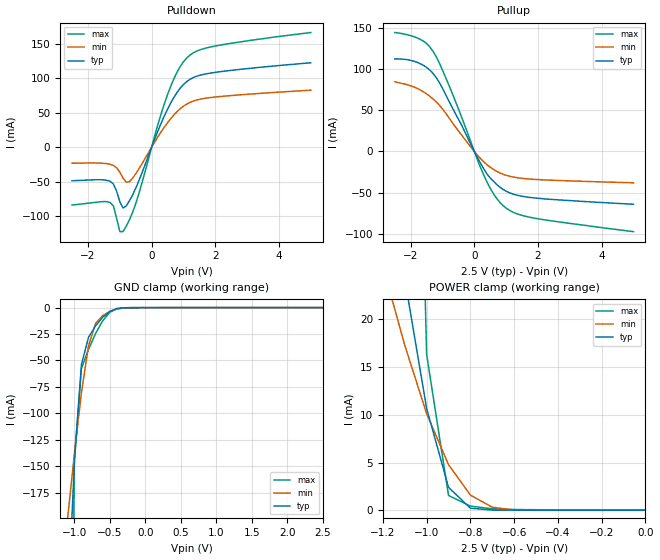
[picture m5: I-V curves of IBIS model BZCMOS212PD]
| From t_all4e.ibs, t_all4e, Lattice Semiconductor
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|   BZCMOS212PD
[Model]   BZCMOS212PD
Model_type   I/O
Polarity   Non-Inverting
Enable   Active-Low
C_comp   2pF   2pF   2pF
Vinl = 0.5
Vinh = 2.64
[Temperature Range]   25.0000   125.0000   -40.0000
[Voltage Range]   2.5000V   2.3000V   2.7000V
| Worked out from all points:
|   slope of the pulldown table from 0 to 0.375 V, typ, clamps not added: 8.75 ohm
|   slope of the pullup table from 0 to 0.375 V, typ, clamps not added: 14.4 ohm
|   GND clamp passes 1 mA (typ) near -0.40 V on its own axis
|   POWER clamp passes 1 mA (typ) near -0.83 V on its own axis
[Pulldown]
|voltage   I(typ)   I(min)   I(max)
-2.5V     -48.8mA    -23.34mA   -84mA
-1.3V     -49.7mA    -24.91mA   -80.43mA
-1.2V     -53.63mA   -26.59mA   -85.64mA
-1V       -79.19mA   -36.36mA   -122.6mA
-900mV    -88.4mA    -44.81mA   -122.7mA
-800mV    -85.34mA   -50.83mA   -115mA
-600mV    -69.53mA   -45.12mA   -94.93mA
500mV     55.24mA    35.55mA    76.37mA
900mV     85.88mA    55.98mA    117.3mA
1.2V      98.44mA    64.96mA    133.6mA
2.1V      109.3mA    73.31mA    147.8mA
5V        122.5mA    82.76mA    166.5mA
[Pullup]
|voltage   I(typ)   I(min)   I(max)
-2.5V     112.7mA    84.9mA     144.8mA
-1.7V     106.9mA    74.88mA    136.5mA
-1.5V     102.3mA    70.1mA     131.4mA
-1.3V     95.06mA    64.02mA    122mA
-1.1V     83.89mA    56.39mA    107.7mA
-700mV    53.9mA     35.54mA    71.28mA
300mV     -21.45mA   -12.87mA   -29.21mA
600mV     -36.24mA   -21.85mA   -51.49mA
900mV     -46.14mA   -27.68mA   -65.82mA
1.3V      -52.82mA   -31.67mA   -75.32mA
1.8V      -56.21mA   -33.75mA   -80.53mA
5V        -64.25mA   -38.14mA   -97.6mA
[GND_clamp]
|voltage   I(typ)   I(min)   I(max)
-2.5V     -2.88A     -1.21A     -25.75A
-1.1V     -296.4mA   -202.8mA   -979.3mA
-1V       -147.6mA   -138.6mA   -143.7mA
-900mV    -53.79mA   -80.42mA   -57.6mA
-800mV    -28.05mA   -35.98mA   -39.41mA
-700mV    -17.1mA    -14.8mA    -24.32mA
-600mV    -8.999mA   -7.523mA   -12.36mA
-500mV    -3.595mA   -3.617mA   -4.359mA
-400mV    -879.6uA   -1.324mA   -818.4uA
-300mV    -134.3uA   -303.2uA   -112.8uA
2.5V      32.9uA     13.5uA     72.78uA
[POWER_clamp]
|voltage   I(typ)   I(min)   I(max)
-2.5V     395.1mA    211mA      2.446A
-1.2V     41.69mA    25.58mA    245.1mA
-1.1V     24.27mA    17.3mA     108.6mA
-1V       10.69mA    10.14mA    16.34mA
-900mV    2.423mA    4.798mA    1.578mA
-800mV    241uA      1.613mA    455.8uA
-700mV    43.59uA    342.3uA    178.8uA
-600mV    33.48uA    49.81uA    99.8uA
0V        32.9uA     13.46uA    72.82uA
[Ramp]
| variable   typ   min   max
dV/dt_r   1.1047/0.9094ns   0.8188/2.3176ns   1.3391/0.2916ns
dV/dt_f   1.2798/0.9412ns   1.0853/2.2217ns   1.4359/0.4171ns
